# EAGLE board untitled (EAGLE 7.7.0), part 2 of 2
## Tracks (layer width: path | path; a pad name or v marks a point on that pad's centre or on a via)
+5V  (2 unrouted)
  Top 0.406: 32.8,2.1 33.2,2.1 33.2,2.2 | T1.E 32.8,2.12 32.8,2.1 | 32.8,2.1 31.5,2.1 31.5,1.2 28.6,1.2 28.6,4.5 25.2,4.5 24,5.7 19.4,5.7 18.6,6.5 18.6,7.8 17.1,9.3
  Top 0.813: R11.2 16.69,10.01 14.6,12.1 13.52,12.1 D1.C
  Top 1.27: C8.1 8.42,19.82 8,19.4 8,18.2 8.8,17.4 10.52,17.4 D1.C
+5V1  (2 unrouted)
  Top 0.406: 32.8,35.4 33.2,35.4 33.2,35.5 | T2.E 32.8,35.42 32.8,35.4 | 32.8,35.4 31.5,35.4 31.5,34.5 28.6,34.5 28.6,37.8 25.2,37.8 24,39 19.4,39 18.6,39.8 18.6,41.1 17.1,42.6
  Top 0.813: R25.2 16.69,43.31 14.6,45.4 13.52,45.4 D3.C
  Top 1.27: C13.1 8.42,53.12 8,52.7 8,51.5 8.8,50.7 10.52,50.7 D3.C
+5V2  (2 unrouted)
  Top 0.406: 32.8,68.7 33.2,68.7 33.2,68.8 | T3.E 32.8,68.72 32.8,68.7 | 32.8,68.7 31.5,68.7 31.5,67.8 28.6,67.8 28.6,71.1 25.2,71.1 24,72.3 19.4,72.3 18.6,73.1 18.6,74.4 17.1,75.9
  Top 0.813: R39.2 16.69,76.61 14.6,78.7 13.52,78.7 D5.C
  Top 1.27: C20.1 8.42,86.42 8,86 8,84.8 8.8,84 10.52,84 D5.C
N$1  (via drill 0.5)  (12 unrouted)
  Top 0.406: 80,13.29 80,13 | Q1.E 22,1.74 22,1.9 | Q1.E 23.34,0.5 40,0.5 40.6,1.1 40.6,2.2 42.1,0.7 75.7,0.7 75.7,1.5 C6.2 | 14.2,16.7 14.4,16.7 14.4,16.3 | Q1.E 21.8,1.4 20.8,0.5 13.1,0.5 11.4,1.9 11.4,7.2 11.2,7.4 4.89,7.4 X1.2
  Top 1.27: 25.4,17.3 25.4,17.5 21.7,17.5 21.7,17.4 21.6,17.4 21.6,17.5 20.8,17.5 20.8,16.2 21.7,16.2 | R5.2 89.2,13.16 89.2,10.6 70.1,10.6 70.1,13.2 69.8,13.2 69.8,10.6 | 69.8,10.5 69.8,10.6 | 69.8,10.6 70.8,10.6 70.8,11.2 71.1,11.2 71.1,12.2 88.6,12.2 88.6,12.1 87.9,12.1 87.9,11.4 71.9,11.4 71.9,11.2 | D1.A 14.16,17.16 C8.2 14.4,19.82 14.4,16.7 | 14.4,16.3 15.2,16.3 v15.8,18.2 | C2.2 21.7,14.63 21.7,16.1 | 21.7,16.2 v21.7,16.7 v23,16.7 U$1.1 | 15.78,16.7 15.78,17.71 | 21.7,16.2 21.7,16.1 | 21.7,16.1 21.4,16.1 21.4,16.9
  Top 3.81: C5.- 68.9,23.37 68.9,24.4
  Bottom 1.27: 39.5,2 19.4,2 19.4,5.4 36.7,5.4 37.8,4.3 37.8,3 37.5,2.7 20.6,2.7 20.2,3.1 20.2,4 20.4,4.2 36.5,4.2 37.2,3.5 21.3,3.5 21.2,3.4 37.1,3.4 39,1.5 20.1,1.5 | 20.1,1.5 19.4,1.5 | 19.4,1.5 19.4,4.8 18.7,5.5 18.7,16.7 | 18.7,16.7 18.7,20.9 17.6,22 12.9,22 10.2,24.7 10.7,24.7 10.7,27.8 10.5,28 10.5,25.8 10.3,25.6 10.3,25.3 13,22.6 16.4,22.6 | 16.4,22.6 18.5,22.6 18.6,22.5 18.6,21.5 18.4,21.3 | 18.4,21.3 18.7,21.3 | 18.4,21.3 12.6,21.3 10.3,23.6 10.3,21.6 10.8,21.6 12,20.4 15,20.4 15.2,20.6 v15.8,18.2 | v15.8,18.2 15.2,1.5 15.3,1.4 20,1.4 20.1,1.5 | 19.4,1.5 18.8,1.5 18.5,1.8 18.5,4.7 18.6,4.8 | v15.8,18.2 15.7,20.1 15.7,18.1 | v21.7,16.7 v20.5,16.7 | v20.5,16.7 18.7,16.7 | C1.- 16.4,28.3 16.4,22.6 | v20.5,16.7 23.6,16.7 23.6,17.9 19.4,17.9
  Bottom 2.54: 85.2,10.7 86.9,10.7 86.9,9.9 89.6,9.9 89.6,24.1 68.3,24.1 68.3,24.7 68.5,24.7 68.5,22 69.6,22 69.6,20.3 69.5,20.3 69.5,14 42.6,14 42.6,14.3 | 42.4,14.3 42.4,11.2 87.9,11.2 87.9,22.7 71.39,22.7 | 69.3,22.7 71.39,22.7 | 71.39,22.7 R5.2 42.8,13.16 42.8,12.8 43.6,12.8 43.6,5.2 71.8,5.2 | 71.8,5.2 71.8,4.9 | 71.8,5.2 71.8,9.3 45.3,9.3 45.3,10.6 45.8,10.6 45.8,6.6 70.7,6.6 70.7,7.3 47,7.3 47,7.8 72.4,7.8 v72.4,11.1 72.4,21.9 85.6,21.9 85.6,20.7 86.5,20.7 86.5,13.7 74.4,13.7 | 74.4,13.7 74.4,12.89 | 74.4,13.7 74.4,20.7 84.9,20.7 84.9,19.1 85.4,19.1 85.4,14.7 75.6,14.7 75.6,14.5 76.1,14.5 76.1,18.6 83.3,18.6 83.3,18.2 83.5,18.2 83.5,16.4 77.9,16.4 77.9,16.2 83.4,16.2 83.4,4.5 80.4,4.5 | 80.4,4.5 80.4,4.3 | 80.4,4.5 80.4,9.3 81.9,9.3 | 82.5,9.3 81.9,9.3 | 81.9,9.3 81.9,4.9 | 84.7,2.6 85.6,2.6 85.6,1.5 78.3,1.5 78.3,2 78.4,2 78.4,3.1 82.5,3.1 82.5,2.6 78.1,2.6 78.1,3.7 39.5,3.7 39.5,2 73.2,2 73.2,2.4 73,2.4 73,2.6 | X1.2 4.46,7.9 7.9,7.9 8.7,8.7 8.7,32 7.2,32 7.7,31.5 7.7,1.2 8.7,1.2 8.8,1.3 8.8,8.1 8.01,8.89 C4.-
  Bottom 3.81: 84.7,2.6 84.7,2.8 85.2,2.8 85.2,10.7
N$2  (3 unrouted)
  Top 1.27: U$1.3 30.4,13.3 30.4,13.6 30.3,13.6 30.2,18.2 30.2,19.7 | DPAK1.1 31.17,27.4 30.4,27.4 30.4,22.6 30.2,22.6 30.2,20.4 30.2,19.7 | PAD4.1 47,18.2 47,19.7 30.2,19.7
N$3  (3 unrouted)
  Top 1.27: R9.2 2.78,27.11 C4.+ 2.93,28.3 2.9,28.3 2.9,32.4 17.8,32.4 17.8,23.12 | U$1.4 21.74,11.6 | 21.74,11.6 C2.1 | 21.74,11.6 17.8,11.6 17.8,23.12 | R14.2 17.8,23.12
  Bottom 1.016: X1.3 3,2.78 3,4.2 5.2,4.2 5.2,0.6 1.6,0.6 | 1.6,0.6 1.6,0.5 | 1.6,0.6 1.6,1.2 4.5,1.2
  Bottom 1.27: L1.1 64.2,18.2 64.2,17.9 64.3,17.9 64.3,31.8 17.8,31.8 17.8,32.1
  Bottom 2.54: X1.3 1.3,2.78 1.3,32.1 3.5,32.1 3.5,16.8
N$4  (4 unrouted)
  Top 0.406: 71.72,15.63 72,15.63 72,16.2 | X2.2 95.9,24.88 95.9,25.1
  Top 1.27: R6.2 71.72,15.63 R5.1
  Top 2.54: X2.2 98.7,24.88 98.7,23.5 98.6,23.5 98.6,16 71.1,16 71.1,16.5 72,16.5 72,16.2
N$5
  Top 0.406: R7.2 R8.1 44.63,5 46.3,5 48.5,2.8 73.1,2.8 75.65,5.35 C6.1
N$6  (2 unrouted)
  Top 0.406: R7.1 44.3,10.74 44.3,10.9 | 45.35,10.85 46.7,9.5 46.7,7.9 50.1,4.5 69.7,4.5 74.3,8 77.1,8 80.05,5.95 80.05,3.75 80.4,3.4 88.8,3.4 | 45.35,10.85 45.3,10.9 | R6.1 92.38,4.48 91.4,3.5 88.9,3.5 | 45.35,10.85 44.51,10.85 R7.1 | U$1.5 25.6,9.9 25.6,5.3 42.9,5.3 42.9,10.3 44.2,10.3 | D2.A 44.51,13.1 R7.1
N$7  (3 unrouted)
  Top 0.406: 79.5,29.96 79.5,30.79 | D2.C 44.6,15.1 57.1,15.1 57.1,32.4
  Top 1.27: DPAK1.4 40,25.3 40,32.4 57.1,32.4 65.4,32.4 65.4,32.5
  Top 3.81: 78.22,31.02 77.6,30.4 77.6,28.79 C5.+
N$8  (1 unrouted)
  Top 0.406: R11.1 16.69,5.5 17.8,5.5 17.8,4.8 23.6,4.8 23.6,3.1 | Q1.C R12.2
N$9
  Top 0.406: T1.B 32.7,4.02 32.7,3.8 29.96,3.8 R12.1
N$10
  Bottom 1.27: 3.9,6.3 7.8,6.3
N$11  (via drill 0.5)
  other vias: 20.5,17.9
N$12  (via drill 0.5)
  other vias: 21.7,17.9
N$13
  Top 0.406: 35.3,2.9 35.3,3.07 T1.C 35.14,2.8 38.2,2.8 | 38.2,2.8 38.2,2.69 R13.2 38.3,2.69 38.3,4.5 42.2,4.5 42.7,4 42.7,2.5 44.33,2.5 R8.2 | 38.2,2.9 38.2,2.8
N$14
  Top 0.406: R10.2 19.3,2.31 19.3,3.8 21.8,3.8 Q1.B
N$15  (1 unrouted)
  Top 0.406: 15.9,2.7 16,2.8 16,3 15.9,3.1 15.9,4.1 15,5 15,8 14.6,8.4 9.4,12.8 9.4,12.84 X1.1
N$16  (3 unrouted)
  Top 1.27: R23.2 2.78,60.41 C10.+ 2.93,61.6 2.9,61.6 2.9,65.7 17.8,65.7 17.8,56.42 | U$2.4 21.74,44.9 | 21.74,44.9 C7.1 | 21.74,44.9 17.8,44.9 17.8,56.42 | R28.2 17.8,56.42
  Bottom 1.016: X3.3 3,36.08 3,37.5 5.2,37.5 5.2,33.9 1.6,33.9 | 1.6,33.9 1.6,33.8 | 1.6,33.9 1.6,34.5 4.5,34.5
  Bottom 1.27: L2.1 64.2,51.5 64.2,51.2 64.3,51.2 64.3,65.1 17.8,65.1 17.8,65.4
  Bottom 2.54: X3.3 1.3,36.08 1.3,65.4 3.5,65.4 3.5,50.1
N$17  (4 unrouted)
  Top 0.406: 71.72,48.93 72,48.93 72,49.5 | X4.2 95.9,58.18 95.9,58.4
  Top 1.27: R20.2 71.72,48.93 R19.1
  Top 2.54: X4.2 98.7,58.18 98.7,56.8 98.6,56.8 98.6,49.3 71.1,49.3 71.1,49.8 72,49.8 72,49.5
N$18  (via drill 0.5)
  other vias: 23,17.9
N$19
  Top 0.406: R21.2 R22.1 44.63,38.3 46.3,38.3 48.5,36.1 73.1,36.1 75.65,38.65 C12.1
N$20  (1 unrouted)
  Top 0.406: R25.1 16.69,38.8 17.8,38.8 17.8,38.1 23.6,38.1 23.6,36.4 | Q2.C R26.2
N$21
  Top 0.406: 35.3,36.2 35.3,36.37 T2.C 35.14,36.1 38.2,36.1 | 38.2,36.1 38.2,35.99 R27.2 38.3,35.99 38.3,37.8 42.2,37.8 42.7,37.3 42.7,35.8 44.33,35.8 R22.2 | 38.2,36.2 38.2,36.1
N$22  (1 unrouted)
  Top 0.406: 15.9,36 16,36.1 16,36.3 15.9,36.4 15.9,37.4 15,38.3 15,41.3 14.6,41.7 9.4,46.1 9.4,46.14 X3.1
N$23
  Top 0.406: R24.2 19.3,35.61 19.3,37.1 21.8,37.1 Q2.B
N$24
  Top 0.406: T2.B 32.7,37.32 32.7,37.1 29.96,37.1 R26.1
N$25
  Top 1.27: 20.4,16.1 20.3,16.1 20.3,17.9 23.1,17.9 | 23.5,17.9 23.1,17.9 | 23.1,17.9 23.1,16 20.4,16
N$26  (via drill 0.5)
  Top 1.27: 18.6,12.2 18.7,12.2 18.7,32.5 2.2,32.5 2.2,32.4 0.7,32.4 0.7,32.2 0.6,32.2 v0.7,31.4 0.6,26.1 4.1,26.1 4.1,26.3 4.2,26.3 4.2,32.6 v3.1,32.6 v1.9,32.6 v0.7,32.6 0.6,32.6 0.6,32.5 1.8,32.5 v1.9,31.4 1.8,26.9
N$27  (via drill 0.5)
  Top 1.27: 4.7,31.4 v15.6,31.4 v16.8,31.4 17.9,31.4 17.9,31.3 17.6,31.3 17.6,30.2 v16.8,30.2 v15.6,30.2 4,30.2 4,30.5
  Bottom 1.27: 63.1,32.4 63.1,32.6 22.2,32.6 | 22.2,32.4 22.2,32.6 | 22.2,32.6 v18,32.6 v16.8,32.6 15.8,32.6 15.8,31.7 15.9,31.7 | 17.5,31.7 15.9,31.7 | 15.9,31.7 15.9,31 63.2,31 | 64.3,17.2 65.3,17.2 65.3,32.6 63.2,32.6 63.2,31 | 63.2,30.8 63.2,17 | 63.2,31 63.2,30.8 | 63.2,30.8 62.7,30.8 62.7,30.1 15.6,30.1 v15.6,30.2 v15.6,31.4 v15.6,32.6
N$28  (via drill 0.5)
  Top 1.27: 63.4,31.1 40.6,31.1 | 40.6,31.1 40.6,31.6 | 40.6,31.1 40.6,29.8 40.7,29.8 | 64.2,29.8 40.7,29.8 | 40.7,29.8 40.7,27.8 39.1,27.8 39.1,27.9 39.2,27.9 39.2,32.4 38.2,32.4 38.2,32.1 38.1,32.1 38.1,27.9 v35,28 33.8,27.9 33.8,32.6 73.7,32.6 73.7,32.5 35,32.5 35,28.8 37.1,28.8 37.1,31.3 36.1,31.3 | 36.1,31.3 36.1,31.4 | 36.1,31.3 36.1,29.6
N$29
  Top 1.27: 33.8,27.6 33.6,27.6 33.6,22.7 | 33.6,22.7 33.6,22.6 | 33.6,22.6 41.8,22.6 41.8,30.2 43,30.2 43,22.4 44.1,22.4 44.1,30.2 45.2,30.2 45.2,22.4 | 45.2,22.4 33.6,22.4 33.6,22.6 | 33.6,22.7 34.6,22.7 34.6,27.1 35.8,27.1 35.8,23.6 36.8,23.6 36.8,27.1 37,27.1 37,25.9 | 45.2,22.4 65.8,22.4 65.8,28.9 69.7,28.9 69.7,28.8 46.2,28.8 46.2,23.4 64.7,23.4 64.7,27.9 47.1,27.9 47.1,28 47.2,28 47.2,24.5 63.7,24.5 | 63.7,24.5 63.7,24.4 | 63.7,24.5 63.7,26.9 48.1,26.9 48.1,25.5 63,25.5 63,26.2 49,26.2 49,26.1
N$30
  Top 1.27: 45.5,30.5 62.8,30.5
N$31
  Top 1.27: 40.9,31.9 63.2,31.9 63.2,32
N$32
  Top 1.27: 31.6,27.3 31.7,27.3 31.7,23.7 31.4,23.7 31.4,18.9 32,18.9 32,27.4 30.9,27.4 30.9,24.6 29.4,24.6 29.4,27.7 29.3,27.7 29.3,18.6 29,18.6 29,27.8 32,27.8 32,27.7
N$33
  Top 1.27: 32.5,20.3 50.5,20.3 | 50.5,20.3 50.5,20.2 | 50.5,20.2 50.5,19.8 47.7,19.8 47.7,19.6 50.6,19.6 50.6,17 50.7,17 50.7,16.7 46.8,16.7 46.8,16.9 46.6,16.9 46.6,18.6 32.9,18.6 32.9,19.6 32.7,19.6 32.7,20.7 50.5,20.7 50.5,20.3 | 50.5,20.2 39.6,20.2 39.6,16.1 39.4,16.1 39.4,8.2 38.9,8.2 38.9,17.8 28.6,17.8 28.6,6.6 41.7,6.6 41.7,18 40.6,18 40.6,7.4 29.5,7.4 29.5,7.5
N$34
  Top 1.27: 19.3,12.2 23.1,12.2 23.1,10.9 18.2,10.9 18.2,11 17.7,11 17.7,11.2 17.6,11.2 17.6,15.2 17.5,15.2 17.5,29.4
N$35
  Top 1.27: 16.6,29.8 16.6,22.1 16.9,22.1 16.9,22.2
N$36
  Top 1.27: 18.6,32.4 18.8,32.4 18.8,32.5
N$37  (via drill 0.5)
  Top 1.27: 32,27.9 32,32.6 25.7,32.6 25.7,27.5 25.8,27.5 25.8,21.7 v27.1,21.7 28.4,21.7 28.4,21.6 26.7,21.6 26.7,31.6 31.1,31.6 31.1,28.9 27.8,28.9 27.8,22.6 28.4,22.6 v28.4,23 v28.4,24.3 v28.4,25.6 v28.4,26.9 v28.4,28.2 28.4,30.7 27.6,30.7 27.6,29.6 30.2,29.6 30.2,29.7 29.2,29.7 29.2,30.7 30.3,30.7 30.3,30.5
N$38  (via drill 0.5)
  other vias: 3.2,31.4
N$39  (via drill 0.5)
  other vias: 0.7,30.2
N$40  (via drill 0.5)
  other vias: 1.9,30.2
N$41  (via drill 0.5)
  other vias: 3.2,30.2
N$42  (via drill 0.5)
  other vias: 33.5,7.1
N$43  (via drill 0.5)
  other vias: 34.7,7.1
N$44  (via drill 0.5)
  other vias: 18,31.4
N$45  (via drill 0.5)
  other vias: 18.1,30.2
N$46  (via drill 0.5)
  other vias: 28.7,7.1
N$47  (via drill 0.5)
  other vias: 29.9,7.1
N$48  (via drill 0.5)
  other vias: 31.1,7.1
N$49  (via drill 0.5)
  other vias: 32.3,7.1
N$50  (via drill 0.5)
  other vias: 35.9,7.1
N$51  (via drill 0.5)
  other vias: 37.1,7.1
N$52  (via drill 0.5)
  other vias: 38.3,7.1
N$53  (via drill 0.5)
  other vias: 39.5,7.1
N$54  (via drill 0.5)
  other vias: 40.7,7.1
N$55  (via drill 0.5)
  other vias: 39.9,8.4
N$56  (via drill 0.5)
  other vias: 41.2,8.4
N$57  (via drill 0.5)
  other vias: 36.2,22.9
N$58  (via drill 0.5)
  other vias: 40.2,11
N$59  (via drill 0.5)
  other vias: 40.2,12.2
N$60  (via drill 0.5)
  other vias: 40.2,13.5
N$61  (via drill 0.5)
  other vias: 40.2,14.8
N$62  (via drill 0.5)
  other vias: 40.2,16.1
N$63  (via drill 0.5)
  other vias: 40.2,17.4
N$64  (via drill 0.5)
  other vias: 29.2,19.3
N$65  (via drill 0.5)
  other vias: 30.4,19.3
N$66  (via drill 0.5)
  other vias: 31.6,19.3
N$67  (via drill 0.5)
  other vias: 32.8,19.3
N$68  (via drill 0.5)
  other vias: 34,19.3
N$69  (via drill 0.5)
  other vias: 35.2,19.3
N$70  (via drill 0.5)
  other vias: 36.4,19.3
N$71  (via drill 0.5)
  other vias: 37.6,19.3
N$72  (via drill 0.5)
  other vias: 38.8,19.3
N$73  (via drill 0.5)
  other vias: 40,19.3
N$74  (via drill 0.5)
  other vias: 29.2,20.5
N$75  (via drill 0.5)
  other vias: 30.4,20.5
N$76  (via drill 0.5)
  other vias: 31.6,20.5
N$77  (via drill 0.5)
  other vias: 32.8,20.5
N$78  (via drill 0.5)
  other vias: 34,20.5
N$79  (via drill 0.5)
  other vias: 35.2,20.5
N$80  (via drill 0.5)
  other vias: 36.4,20.5
N$81  (via drill 0.5)
  other vias: 37.6,20.5
N$82  (via drill 0.5)
  other vias: 38.8,20.5
N$83
  Top 2.54: 71.4,16.8 96.2,16.8 96.2,25.1 87.3,25.1 87.3,24.9 87.5,24.9 87.5,18.7 94.3,18.7 | 94.5,18.7 94.3,18.7 | 94.3,18.7 94.3,23.3 89.7,23.3 89.7,20.1 93.1,20.1 93.1,20.3 91.9,20.3 91.9,21.7
N$84
  Top 3.81: 88.3,30.7 97.9,30.7 97.9,31 88.4,31 88.4,31.1 64.7,31.1 64.7,31.2
N$85
  Top 2.54: 71.4,50.1 96.2,50.1 96.2,58.4 87.3,58.4 87.3,58.2 87.5,58.2 87.5,52 94.3,52 | 94.5,52 94.3,52 | 94.3,52 94.3,56.6 89.7,56.6 89.7,53.4 93.1,53.4 93.1,53.6 91.9,53.6 91.9,55
N$86
  Top 3.81: 88.3,64 97.9,64 97.9,64.3 88.4,64.3 88.4,64.4 64.7,64.4 64.7,64.5
N$87
  Bottom 2.54: 72.9,41.2 72.9,38.8 72.8,38.8 72.8,43.1 78.4,43.1 78.4,38.6
N$88  (via drill 0.5)
  other vias: 88.1,44.4
N$89  (via drill 0.5)
  other vias: 86.9,44.4
N$90  (via drill 0.5)
  other vias: 85.7,44.4
N$91  (via drill 0.5)
  other vias: 84.5,44.4
N$92  (via drill 0.5)
  other vias: 83.3,44.4
N$93
  Bottom 2.54: 72.9,7.9 72.9,5.5 72.8,5.5 72.8,9.8 78.4,9.8 78.4,5.3
N$94  (via drill 0.5)
  other vias: 88.1,11.1
N$95  (via drill 0.5)
  other vias: 86.9,11.1
N$96  (via drill 0.5)
  other vias: 85.7,11.1
N$97  (via drill 0.5)
  other vias: 84.5,11.1
N$98  (via drill 0.5)
  other vias: 83.3,11.1
N$99  (via drill 0.5)
  other vias: 82.1,11.1
N$100  (via drill 0.5)
  other vias: 80.9,11.1
N$101  (via drill 0.5)
  other vias: 79.7,11.1
N$102  (via drill 0.5)
  other vias: 78.5,11.1
N$103  (via drill 0.5)
  other vias: 77.3,11.1
N$104  (via drill 0.5)
  other vias: 76,11.1
N$105  (via drill 0.5)
  other vias: 74.8,11.1
N$106  (via drill 0.5)
  other vias: 73.6,11.1
N$107  (via drill 0.5)
  other vias: 71.2,11.1
N$108  (via drill 0.5)
  other vias: 69.9,11.1
N$109  (via drill 0.5)
  other vias: 67.9,23.6
N$110  (via drill 0.5)
  other vias: 69.2,23.6
N$111  (via drill 0.5)
  other vias: 70.5,23.6
N$112  (via drill 0.5)
  other vias: 71.8,23.6
N$113  (via drill 0.5)
  other vias: 73.1,23.6
N$114  (via drill 0.5)
  other vias: 74.4,23.6
N$115  (via drill 0.5)
  other vias: 74.4,22.3
N$116  (via drill 0.5)
  other vias: 73.1,22.3
N$117  (via drill 0.5)
  other vias: 71.7,22.3
N$118  (via drill 0.5)
  other vias: 70.4,22.3
N$119  (via drill 0.5)
  other vias: 69.1,22.3
N$120  (via drill 0.5)
  other vias: 67.9,22.4
N$121  (via drill 0.5)
  other vias: 82.1,44.4
N$122  (via drill 0.5)
  other vias: 80.9,44.4
N$123  (via drill 0.5)
  other vias: 79.7,44.4
N$124  (via drill 0.5)
  other vias: 78.5,44.4
N$125  (via drill 0.5)
  other vias: 77.3,44.4
N$126  (via drill 0.5)
  other vias: 76,44.4
N$127  (via drill 0.5)
  other vias: 74.8,44.4
N$128  (via drill 0.5)
  other vias: 73.6,44.4
N$129  (via drill 0.5)
  other vias: 40,20.6
N$130
  Bottom 1.27: 18.1,2.2 16,2.2 16,20.7 | 16,20.7 16.7,20.7 | 16.7,20.7 17.8,20.7 17.8,2.9 17,2.9 17,3.1 16.8,3.1 16.8,20.4 16.7,20.4 16.7,20.7 | 16,20.7 10.3,20.7 10.3,25.1 10.2,25.1 10.2,28 9.8,28 9.8,25.6
N$131
  Top 1.27: 14.6,16 15.8,16 15.8,20.1 15.1,20.1 | 15,20.1 15.1,20.1 | 15.1,20.1 15.1,17.6 14.2,17.6 14.2,16
N$132  (via drill 0.5)
  other vias: 71.2,44.4
N$133  (via drill 0.5)
  other vias: 41.2,20.5
N$134  (4 unrouted)
  Top 0.406: 25.9,14.9 25.9,15 27.1,15 27.1,20.28 R14.1 24,20.28 24,28.2
  Top 1.27: U$1.2 25.1,15
N$135  (via drill 0.5)
  other vias: 41.2,19.3
N$136  (via drill 0.5)
  other vias: 41.4,17.8
N$137  (via drill 0.5)
  other vias: 41.5,16.5
N$138  (via drill 0.5)
  other vias: 28.4,21.8
N$139  (via drill 0.5)
  other vias: 27.1,28.2
N$140  (via drill 0.5)
  other vias: 27.1,27
N$141  (via drill 0.5)
  other vias: 27.1,25.6
N$142  (via drill 0.5)
  other vias: 27.1,24.3
N$143  (via drill 0.5)
  other vias: 27.1,22.9
N$144  (via drill 0.5)
  other vias: 42.5,22.7
N$145  (via drill 0.5)
  other vias: 42.5,24
N$146  (via drill 0.5)
  other vias: 42.5,25.3
N$147  (via drill 0.5)
  other vias: 42.5,26.6
N$148  (via drill 0.5)
  other vias: 42.5,27.9
N$149  (via drill 0.5)
  other vias: 43.8,27.9
N$150  (via drill 0.5)
  other vias: 69.9,44.4
N$151  (via drill 0.5)
  other vias: 43.8,26.6
N$152  (via drill 0.5)
  other vias: 43.7,25.3
N$153  (via drill 0.5)
  other vias: 43.7,24
N$154  (via drill 0.5)
  other vias: 43.7,22.7
N$155  (via drill 0.5)
  Bottom 1.27: 34,28.4 v37.5,28.4 v38.7,28.4 v40.1,28.4 v41.3,28.4 61.4,28.4 61.4,22.4 33.9,22.4 33.9,28.4 34.7,28.4 34.7,23
N$156
  Bottom 1.27: 35.3,23.2 60.6,23.2 60.6,27.4 35.6,27.4 35.6,24.3 59.7,24.3 59.7,26.5 36.6,26.5 36.6,25.3
N$157
  Bottom 1.27: 37.3,25.2 59.2,25.2 59.2,25.5 37.6,25.5 37.6,26.2
N$158  (via drill 0.5)
  Bottom 1.27: 25.8,28.2 25.7,28.2 | 25.7,28.2 25.7,28.3 | 25.7,28.3 25.7,28.5 32,28.5 32,20.2 32.8,20.2 32.8,20.7 50.5,20.7 50.5,20.4 50.6,20.4 50.6,16.7 41.7,16.7 41.7,17.5 41.4,17.5 41.4,19.9 49.7,19.9 49.7,19.4 42.7,19.4 42.7,17.5 49.6,17.5 49.6,18.6 43.7,18.6 43.7,18.5 40.5,18.5 40.5,15.8 40.3,15.8 40.3,15.1 40.1,15.1 v40.1,9.7 40.1,8.9 41.3,8.9 41.3,7.1 25.7,7.1 25.7,28.2 | 25.7,28.3 31,28.3 31,20.1 26.3,20.1 26.3,20.8 26.5,20.8 26.5,27.7 30.1,27.7 30.1,21.1 27.4,21.1 27.4,27.2 29,27.2 29,21.6 28.1,21.6 28.1,26.5
N$159
  Bottom 1.27: 26.4,19.1 40.8,19.1 40.8,19.9 34,19.9 34,19.8 39.3,19.8 39.3,7.3 40.3,7.3 40.3,7.9 26.8,7.9 26.8,18.2 39,18.2 39,8.4 27.5,8.4 27.5,17.3 37.9,17.3 37.9,9.1 28.5,9.1 28.5,16.3 36.8,16.3 36.8,10 29.4,10 29.4,15.4 35.6,15.4 35.6,10.8 30.3,10.8 30.3,14.7 34.5,14.7 34.5,11.8 31.3,11.8 31.3,13.7 33.5,13.7 33.5,12.6 32.2,12.6 32.2,12.8
N$160
  Bottom 1.27: 37.5,5 43,5 43,5.1 42.5,5.1 | 42.5,5.1 37,5.1 | 37,5.1 37,5.3 42.5,5.3 42.5,5.1 | 37,5.1 19.3,5.1 19.3,23 12.1,23 12.1,22.9
N$161
  Top 0.406: 23.6,28.3 23.7,28.3 23.7,20.6 22.8,20.6
N$162
  Bottom 0.406: 25.6,6.7 20.5,6.7 20.5,15.3 25.1,15.3 25.1,7 20.8,7 20.8,15.1 24.8,15.1 24.8,14.8 24.7,14.8 24.7,7.3 21.2,7.3 21.2,7.4 21,7.4 21,14.9 24.4,14.9 24.4,7.7 21.3,7.7 21.3,14.7 24,14.7 24,8 21.6,8 21.6,14.5 23.7,14.5 23.7,8.3 21.9,8.3 21.9,14.3 23.4,14.3 23.4,8.4 22.3,8.4 22.3,14 23.1,14 23.1,8.7 22.7,8.7 22.7,13.8 22.4,13.8 22.4,13.1
N$163
  Bottom 0.406: 25.3,19.3 25,19.3 25,15.6 24.9,15.6 24.9,19.2 20.6,19.2 20.6,20 20.7,20 20.7,26.6 25.1,26.6 25.1,26.1 24.9,26.1 24.9,26.4 25,26.4 25,19.5 20.9,19.5 20.9,19.8 21,19.8 21,26.2 24.7,26.2 24.7,19.8 21.3,19.8 21.3,25.8 24.4,25.8 24.4,20.1 21.7,20.1 21.7,25.5 24,25.5 24,20.3 22.1,20.3 22.1,25.2 23.7,25.2 23.7,20.6 22.5,20.6 22.5,24.9 23.4,24.9 23.4,20.8 22.9,20.8 22.9,24.6
N$164  (via drill 0.5)
  other vias: 36.2,24.2
N$165  (via drill 0.5)
  other vias: 36.2,25.5
N$166  (via drill 0.5)
  other vias: 36.3,26.7
N$167  (via drill 0.5)
  other vias: 36.3,28
N$168  (via drill 0.5)
  other vias: 34.8,22.9
N$169  (via drill 0.5)
  other vias: 34.8,24.2
N$170  (via drill 0.5)
  other vias: 34.9,25.5
N$171  (via drill 0.5)
  other vias: 35,26.7
N$172  (via drill 0.5)
  other vias: 67.9,56.9
N$173  (via drill 0.5)
  other vias: 69.2,56.9
N$174  (via drill 0.5)
  other vias: 70.5,56.9
N$175  (via drill 0.5)
  other vias: 71.8,56.9
N$176  (via drill 0.5)
  other vias: 73.1,56.9
N$177  (via drill 0.5)
  other vias: 74.4,56.9
N$178  (via drill 0.5)
  other vias: 74.4,55.6
N$179  (via drill 0.5)
  other vias: 73.1,55.6
N$180  (via drill 0.5)
  other vias: 71.7,55.6
N$181  (via drill 0.5)
  other vias: 70.4,55.6
N$182  (via drill 0.5)
  other vias: 69.1,55.6
N$183  (via drill 0.5)
  other vias: 67.9,55.7
N$184
  Bottom 1.27: 3.9,39.6 7.8,39.6
N$185
  Bottom 1.27: 18.1,35.5 16,35.5 16,54 | 16,54 16.7,54 | 16.7,54 17.8,54 17.8,36.2 17,36.2 17,36.4 16.8,36.4 16.8,53.7 16.7,53.7 16.7,54 | 16,54 10.3,54 10.3,58.4 10.2,58.4 10.2,61.3 9.8,61.3 9.8,58.9
N$186
  Top 1.27: 14.6,49.3 15.8,49.3 15.8,53.4 15.1,53.4 | 15,53.4 15.1,53.4 | 15.1,53.4 15.1,50.9 14.2,50.9 14.2,49.3
N$187  (3 unrouted)
  Top 1.27: U$2.3 30.4,46.6 30.4,46.9 30.3,46.9 30.2,51.5 30.2,53 | DPAK2.1 31.17,60.7 30.4,60.7 30.4,55.9 30.2,55.9 30.2,53.7 30.2,53 | PAD2.1 47,51.5 47,53 30.2,53
N$188  (4 unrouted)
  Top 0.406: 25.9,48.2 25.9,48.3 27.1,48.3 27.1,53.58 R28.1 24,53.58 24,61.5
  Top 1.27: U$2.2 25.1,48.3
N$189  (3 unrouted)
  Top 0.406: X4.1 79.5,63.26 79.5,64.09 | D4.C 44.6,48.4 57.1,48.4 57.1,65.7
  Top 1.27: DPAK2.4 40,58.6 40,65.7 57.1,65.7 65.4,65.7 65.4,65.8
  Top 3.81: 78.22,64.32 77.6,63.7 77.6,62.09 C11.+
N$190  (2 unrouted)
  Top 0.406: R21.1 44.3,44.04 44.3,44.2 | 45.35,44.15 46.7,42.8 46.7,41.2 50.1,37.8 69.7,37.8 74.3,41.3 77.1,41.3 80.05,39.25 80.05,37.05 80.4,36.7 88.8,36.7 | 45.35,44.15 45.3,44.2 | R20.1 92.38,37.78 91.4,36.8 88.9,36.8 | 45.35,44.15 44.51,44.15 R21.1 | U$2.5 25.6,43.2 25.6,38.6 42.9,38.6 42.9,43.6 44.2,43.6 | D4.A 44.51,46.4 R21.1
N$191  (via drill 0.5)  (12 unrouted)
  Top 0.406: 80,46.59 80,46.3 | Q2.E 22,35.04 22,35.2 | Q2.E 23.34,33.8 40,33.8 40.6,34.4 40.6,35.5 42.1,34 75.7,34 75.7,34.8 C12.2 | 14.2,50 14.4,50 14.4,49.6 | Q2.E 21.8,34.7 20.8,33.8 13.1,33.8 11.4,35.2 11.4,40.5 11.2,40.7 4.89,40.7 X3.2
  Top 1.27: 25.4,50.6 25.4,50.8 21.7,50.8 21.7,50.7 21.6,50.7 21.6,50.8 20.8,50.8 20.8,49.5 21.7,49.5 | R19.2 89.2,46.46 89.2,43.9 70.1,43.9 70.1,46.5 69.8,46.5 69.8,43.9 | 69.8,43.8 69.8,43.9 | 69.8,43.9 70.8,43.9 70.8,44.5 71.1,44.5 71.1,45.5 88.6,45.5 88.6,45.4 87.9,45.4 87.9,44.7 71.9,44.7 71.9,44.5 | D3.A 14.16,50.46 C13.2 14.4,53.12 14.4,50 | 14.4,49.6 15.2,49.6 v15.8,51.5 | C7.2 21.7,47.93 21.7,49.4 | 21.7,49.5 v21.7,50 v23,50 U$2.1 | 15.78,50 15.78,51.01 | 21.7,49.5 21.7,49.4 | 21.7,49.4 21.4,49.4 21.4,50.2
  Top 3.81: C11.- 68.9,56.67 68.9,57.7
  Bottom 1.27: 39.5,35.3 19.4,35.3 19.4,38.7 36.7,38.7 37.8,37.6 37.8,36.3 37.5,36 20.6,36 20.2,36.4 20.2,37.3 20.4,37.5 36.5,37.5 37.2,36.8 21.3,36.8 21.2,36.7 37.1,36.7 39,34.8 20.1,34.8 | 20.1,34.8 19.4,34.8 | 19.4,34.8 19.4,38.1 18.7,38.8 18.7,50 | 18.7,50 18.7,54.2 17.6,55.3 12.9,55.3 10.2,58 10.7,58 10.7,61.1 10.5,61.3 10.5,59.1 10.3,58.9 10.3,58.6 13,55.9 16.4,55.9 | 16.4,55.9 18.5,55.9 18.6,55.8 18.6,54.8 18.4,54.6 | 18.4,54.6 18.7,54.6 | 18.4,54.6 12.6,54.6 10.3,56.9 10.3,54.9 10.8,54.9 12,53.7 15,53.7 15.2,53.9 v15.8,51.5 | v15.8,51.5 15.2,34.8 15.3,34.7 20,34.7 20.1,34.8 | 19.4,34.8 18.8,34.8 18.5,35.1 18.5,38 18.6,38.1 | v15.8,51.5 15.7,53.4 15.7,51.4 | v21.7,50 v20.5,50 | v20.5,50 18.7,50 | C14.- 16.4,61.6 16.4,55.9 | v20.5,50 23.6,50 23.6,51.2 19.4,51.2
  Bottom 2.54: 85.2,44 86.9,44 86.9,43.2 89.6,43.2 89.6,57.4 68.3,57.4 68.3,58 68.5,58 68.5,55.3 69.6,55.3 69.6,53.6 69.5,53.6 69.5,47.3 42.6,47.3 42.6,47.6 | 42.4,47.6 42.4,44.5 87.9,44.5 87.9,56 71.39,56 | 69.3,56 71.39,56 | 71.39,56 R19.2 42.8,46.46 42.8,46.1 43.6,46.1 43.6,38.5 71.8,38.5 | 71.8,38.5 71.8,38.2 | 71.8,38.5 71.8,42.6 45.3,42.6 45.3,43.9 45.8,43.9 45.8,39.9 70.7,39.9 70.7,40.6 47,40.6 47,41.1 72.4,41.1 v72.4,44.4 72.4,55.2 85.6,55.2 85.6,54 86.5,54 86.5,47 74.4,47 | 74.4,47 74.4,46.19 | 74.4,47 74.4,54 84.9,54 84.9,52.4 85.4,52.4 85.4,48 75.6,48 75.6,47.8 76.1,47.8 76.1,51.9 83.3,51.9 83.3,51.5 83.5,51.5 83.5,49.7 77.9,49.7 77.9,49.5 83.4,49.5 83.4,37.8 80.4,37.8 | 80.4,37.8 80.4,37.6 | 80.4,37.8 80.4,42.6 81.9,42.6 | 82.5,42.6 81.9,42.6 | 81.9,42.6 81.9,38.2 | 84.7,35.9 85.6,35.9 85.6,34.8 78.3,34.8 78.3,35.3 78.4,35.3 78.4,36.4 82.5,36.4 82.5,35.9 78.1,35.9 78.1,37 39.5,37 39.5,35.3 73.2,35.3 73.2,35.7 73,35.7 73,35.9
  Bottom 3.81: 84.7,35.9 84.7,36.1 85.2,36.1 85.2,44
N$192  (via drill 0.5)
  other vias: 20.5,51.2
N$193  (via drill 0.5)
  other vias: 21.7,51.2
N$194  (via drill 0.5)
  other vias: 23,51.2
N$195
  Top 1.27: 20.4,49.4 20.3,49.4 20.3,51.2 23.1,51.2 | 23.5,51.2 23.1,51.2 | 23.1,51.2 23.1,49.3 20.4,49.3
N$196  (via drill 0.5)
  Top 1.27: 18.6,45.5 18.7,45.5 18.7,65.8 2.2,65.8 2.2,65.7 0.7,65.7 0.7,65.5 0.6,65.5 v0.7,64.7 0.6,59.4 4.1,59.4 4.1,59.6 4.2,59.6 4.2,65.9 v3.1,65.9 v1.9,65.9 v0.7,65.9 0.6,65.9 0.6,65.8 1.8,65.8 v1.9,64.7 1.8,60.2
N$197  (via drill 0.5)
  Top 1.27: 4.7,64.7 v15.6,64.7 v16.8,64.7 17.9,64.7 17.9,64.6 17.6,64.6 17.6,63.5 v16.8,63.5 v15.6,63.5 4,63.5 4,63.8
  Bottom 1.27: 63.1,65.7 63.1,65.9 22.2,65.9 | 22.2,65.7 22.2,65.9 | 22.2,65.9 v18,65.9 v16.8,65.9 15.8,65.9 15.8,65 15.9,65 | 17.5,65 15.9,65 | 15.9,65 15.9,64.3 63.2,64.3 | 64.3,50.5 65.3,50.5 65.3,65.9 63.2,65.9 63.2,64.3 | 63.2,64.1 63.2,50.3 | 63.2,64.3 63.2,64.1 | 63.2,64.1 62.7,64.1 62.7,63.4 15.6,63.4 v15.6,63.5 v15.6,64.7 v15.6,65.9
N$198  (via drill 0.5)
  Top 1.27: 63.4,64.4 40.6,64.4 | 40.6,64.4 40.6,64.9 | 40.6,64.4 40.6,63.1 40.7,63.1 | 64.2,63.1 40.7,63.1 | 40.7,63.1 40.7,61.1 39.1,61.1 39.1,61.2 39.2,61.2 39.2,65.7 38.2,65.7 38.2,65.4 38.1,65.4 38.1,61.2 v35,61.3 33.8,61.2 33.8,65.9 73.7,65.9 73.7,65.8 35,65.8 35,62.1 37.1,62.1 37.1,64.6 36.1,64.6 | 36.1,64.6 36.1,64.7 | 36.1,64.6 36.1,62.9
N$199
  Top 1.27: 33.8,60.9 33.6,60.9 33.6,56 | 33.6,56 33.6,55.9 | 33.6,55.9 41.8,55.9 41.8,63.5 43,63.5 43,55.7 44.1,55.7 44.1,63.5 45.2,63.5 45.2,55.7 | 45.2,55.7 33.6,55.7 33.6,55.9 | 33.6,56 34.6,56 34.6,60.4 35.8,60.4 35.8,56.9 36.8,56.9 36.8,60.4 37,60.4 37,59.2 | 45.2,55.7 65.8,55.7 65.8,62.2 69.7,62.2 69.7,62.1 46.2,62.1 46.2,56.7 64.7,56.7 64.7,61.2 47.1,61.2 47.1,61.3 47.2,61.3 47.2,57.8 63.7,57.8 | 63.7,57.8 63.7,57.7 | 63.7,57.8 63.7,60.2 48.1,60.2 48.1,58.8 63,58.8 63,59.5 49,59.5 49,59.4
N$200
  Top 1.27: 45.5,63.8 62.8,63.8
N$201
  Top 1.27: 40.9,65.2 63.2,65.2 63.2,65.3
N$202
  Top 1.27: 31.6,60.6 31.7,60.6 31.7,57 31.4,57 31.4,52.2 32,52.2 32,60.7 30.9,60.7 30.9,57.9 29.4,57.9 29.4,61 29.3,61 29.3,51.9 29,51.9 29,61.1 32,61.1 32,61
N$203
  Top 1.27: 32.5,53.6 50.5,53.6 | 50.5,53.6 50.5,53.5 | 50.5,53.5 50.5,53.1 47.7,53.1 47.7,52.9 50.6,52.9 50.6,50.3 50.7,50.3 50.7,50 46.8,50 46.8,50.2 46.6,50.2 46.6,51.9 32.9,51.9 32.9,52.9 32.7,52.9 32.7,54 50.5,54 50.5,53.6 | 50.5,53.5 39.6,53.5 39.6,49.4 39.4,49.4 39.4,41.5 38.9,41.5 38.9,51.1 28.6,51.1 28.6,39.9 41.7,39.9 41.7,51.3 40.6,51.3 40.6,40.7 29.5,40.7 29.5,40.8
N$204
  Top 1.27: 19.3,45.5 23.1,45.5 23.1,44.2 18.2,44.2 18.2,44.3 17.7,44.3 17.7,44.5 17.6,44.5 17.6,48.5 17.5,48.5 17.5,62.7
N$205
  Top 1.27: 16.6,63.1 16.6,55.4 16.9,55.4 16.9,55.5
N$206
  Top 1.27: 18.6,65.7 18.8,65.7 18.8,65.8
N$207  (via drill 0.5)
  Top 1.27: 32,61.2 32,65.9 25.7,65.9 25.7,60.8 25.8,60.8 25.8,55 v27.1,55 28.4,55 28.4,54.9 26.7,54.9 26.7,64.9 31.1,64.9 31.1,62.2 27.8,62.2 27.8,55.9 28.4,55.9 v28.4,56.3 v28.4,57.6 v28.4,58.9 v28.4,60.2 v28.4,61.5 28.4,64 27.6,64 27.6,62.9 30.2,62.9 30.2,63 29.2,63 29.2,64 30.3,64 30.3,63.8
N$208  (via drill 0.5)
  other vias: 3.2,64.7
N$209  (via drill 0.5)
  other vias: 0.7,63.5
N$210  (via drill 0.5)
  other vias: 1.9,63.5
N$211  (via drill 0.5)
  other vias: 3.2,63.5
N$212  (via drill 0.5)
  other vias: 18,64.7
N$213  (via drill 0.5)
  other vias: 18.1,63.5
N$214  (via drill 0.5)
  other vias: 28.7,40.4
N$215  (via drill 0.5)
  other vias: 29.9,40.4
N$216  (via drill 0.5)
  other vias: 31.1,40.4
N$217  (via drill 0.5)
  other vias: 32.3,40.4
N$218  (via drill 0.5)
  other vias: 33.5,40.4
N$219  (via drill 0.5)
  other vias: 34.7,40.4
N$220  (via drill 0.5)
  other vias: 35.9,40.4
N$221  (via drill 0.5)
  other vias: 37.1,40.4
N$222  (via drill 0.5)
  other vias: 38.3,40.4
N$223  (via drill 0.5)
  other vias: 39.5,40.4
N$224  (via drill 0.5)
  other vias: 40.7,40.4
N$225  (via drill 0.5)
  other vias: 39.9,41.7
N$226  (via drill 0.5)
  other vias: 41.2,41.7
N$227  (via drill 0.5)
  other vias: 40.2,44.3
N$228  (via drill 0.5)
  other vias: 40.2,45.5
N$229  (via drill 0.5)
  other vias: 40.2,46.8
N$230  (via drill 0.5)
  other vias: 40.2,48.1
N$231  (via drill 0.5)
  other vias: 40.2,49.4
N$232  (via drill 0.5)
  other vias: 40.2,50.7
N$233  (via drill 0.5)
  other vias: 29.2,52.6
N$234  (via drill 0.5)
  other vias: 30.4,52.6
N$235  (via drill 0.5)
  other vias: 31.6,52.6
N$236  (via drill 0.5)
  other vias: 32.8,52.6
N$237  (via drill 0.5)
  other vias: 34,52.6
N$238  (via drill 0.5)
  other vias: 35.2,52.6
N$239  (via drill 0.5)
  other vias: 36.4,52.6
N$240  (via drill 0.5)
  other vias: 37.6,52.6
N$241  (via drill 0.5)
  other vias: 38.8,52.6
N$242  (via drill 0.5)
  other vias: 40,52.6
N$243  (via drill 0.5)
  other vias: 29.2,53.8
N$244  (via drill 0.5)
  other vias: 30.4,53.8
N$245  (via drill 0.5)
  other vias: 31.6,53.8
N$246  (via drill 0.5)
  other vias: 32.8,53.8
N$247  (via drill 0.5)
  other vias: 34,53.8
N$248  (via drill 0.5)
  other vias: 35.2,53.8
N$249  (via drill 0.5)
  other vias: 36.4,53.8
N$250  (via drill 0.5)
  other vias: 37.6,53.8
N$251  (via drill 0.5)
  other vias: 38.8,53.8
N$252  (via drill 0.5)
  other vias: 40,53.9
N$253  (via drill 0.5)
  other vias: 41.2,53.8
N$254  (via drill 0.5)
  other vias: 41.2,52.6
N$255  (via drill 0.5)
  other vias: 41.4,51.1
N$256  (via drill 0.5)
  other vias: 41.5,49.8
N$257  (via drill 0.5)
  other vias: 28.4,55.1
N$258  (via drill 0.5)
  other vias: 27.1,61.5
N$259  (via drill 0.5)
  other vias: 27.1,60.3
N$260  (via drill 0.5)
  other vias: 27.1,58.9
N$261  (via drill 0.5)
  other vias: 27.1,57.6
N$262  (via drill 0.5)
  other vias: 27.1,56.2
N$263  (via drill 0.5)
  other vias: 42.5,56
N$264  (via drill 0.5)
  other vias: 42.5,57.3
N$265  (via drill 0.5)
  other vias: 42.5,58.6
N$266  (via drill 0.5)
  other vias: 42.5,59.9
N$267  (via drill 0.5)
  other vias: 42.5,61.2
N$268  (via drill 0.5)
  other vias: 43.8,61.2
N$269  (via drill 0.5)
  other vias: 43.8,59.9
N$270  (via drill 0.5)
  other vias: 43.7,58.6
N$271  (via drill 0.5)
  other vias: 43.7,57.3
N$272  (via drill 0.5)
  other vias: 43.7,56
N$273  (via drill 0.5)
  Bottom 1.27: 34,61.7 v37.5,61.7 v38.7,61.7 v40.1,61.7 v41.3,61.7 61.4,61.7 61.4,55.7 33.9,55.7 33.9,61.7 34.7,61.7 34.7,56.3
N$274
  Bottom 1.27: 35.3,56.5 60.6,56.5 60.6,60.7 35.6,60.7 35.6,57.6 59.7,57.6 59.7,59.8 36.6,59.8 36.6,58.6
N$275
  Bottom 1.27: 37.3,58.5 59.2,58.5 59.2,58.8 37.6,58.8 37.6,59.5
N$276  (via drill 0.5)
  Bottom 1.27: 25.8,61.5 25.7,61.5 | 25.7,61.5 25.7,61.6 | 25.7,61.6 25.7,61.8 32,61.8 32,53.5 32.8,53.5 32.8,54 50.5,54 50.5,53.7 50.6,53.7 50.6,50 41.7,50 41.7,50.8 41.4,50.8 41.4,53.2 49.7,53.2 49.7,52.7 42.7,52.7 42.7,50.8 49.6,50.8 49.6,51.9 43.7,51.9 43.7,51.8 40.5,51.8 40.5,49.1 40.3,49.1 40.3,48.4 40.1,48.4 v40.1,43 40.1,42.2 41.3,42.2 41.3,40.4 25.7,40.4 25.7,61.5 | 25.7,61.6 31,61.6 31,53.4 26.3,53.4 26.3,54.1 26.5,54.1 26.5,61 30.1,61 30.1,54.4 27.4,54.4 27.4,60.5 29,60.5 29,54.9 28.1,54.9 28.1,59.8
N$277
  Bottom 1.27: 26.4,52.4 40.8,52.4 40.8,53.2 34,53.2 34,53.1 39.3,53.1 39.3,40.6 40.3,40.6 40.3,41.2 26.8,41.2 26.8,51.5 39,51.5 39,41.7 27.5,41.7 27.5,50.6 37.9,50.6 37.9,42.4 28.5,42.4 28.5,49.6 36.8,49.6 36.8,43.3 29.4,43.3 29.4,48.7 35.6,48.7 35.6,44.1 30.3,44.1 30.3,48 34.5,48 34.5,45.1 31.3,45.1 31.3,47 33.5,47 33.5,45.9 32.2,45.9 32.2,46.1
N$278
  Bottom 1.27: 37.5,38.3 43,38.3 43,38.4 42.5,38.4 | 42.5,38.4 37,38.4 | 37,38.4 37,38.6 42.5,38.6 42.5,38.4 | 37,38.4 19.3,38.4 19.3,56.3 12.1,56.3 12.1,56.2
N$279
  Top 0.406: 23.6,61.6 23.7,61.6 23.7,53.9 22.8,53.9
N$280
  Bottom 0.406: 25.6,40 20.5,40 20.5,48.6 25.1,48.6 25.1,40.3 20.8,40.3 20.8,48.4 24.8,48.4 24.8,48.1 24.7,48.1 24.7,40.6 21.2,40.6 21.2,40.7 21,40.7 21,48.2 24.4,48.2 24.4,41 21.3,41 21.3,48 24,48 24,41.3 21.6,41.3 21.6,47.8 23.7,47.8 23.7,41.6 21.9,41.6 21.9,47.6 23.4,47.6 23.4,41.7 22.3,41.7 22.3,47.3 23.1,47.3 23.1,42 22.7,42 22.7,47.1 22.4,47.1 22.4,46.4
N$281
  Bottom 0.406: 25.3,52.6 25,52.6 25,48.9 24.9,48.9 24.9,52.5 20.6,52.5 20.6,53.3 20.7,53.3 20.7,59.9 25.1,59.9 25.1,59.4 24.9,59.4 24.9,59.7 25,59.7 25,52.8 20.9,52.8 20.9,53.1 21,53.1 21,59.5 24.7,59.5 24.7,53.1 21.3,53.1 21.3,59.1 24.4,59.1 24.4,53.4 21.7,53.4 21.7,58.8 24,58.8 24,53.6 22.1,53.6 22.1,58.5 23.7,58.5 23.7,53.9 22.5,53.9 22.5,58.2 23.4,58.2 23.4,54.1 22.9,54.1 22.9,57.9
N$282  (via drill 0.5)
  other vias: 36.2,56.2
N$283  (via drill 0.5)
  other vias: 36.2,57.5
N$284  (via drill 0.5)
  other vias: 36.2,58.8
N$285  (via drill 0.5)
  other vias: 36.3,60
N$286  (via drill 0.5)
  other vias: 36.3,61.3
N$287  (via drill 0.5)
  other vias: 34.8,56.2
N$288  (via drill 0.5)
  other vias: 34.8,57.5
N$289  (via drill 0.5)
  other vias: 34.9,58.8
N$290  (via drill 0.5)
  other vias: 35,60
N$291  (3 unrouted)
  Top 1.27: R37.2 2.78,93.71 C17.+ 2.93,94.9 2.9,94.9 2.9,99 17.8,99 17.8,89.72 | U$3.4 21.74,78.2 | 21.74,78.2 C15.1 | 21.74,78.2 17.8,78.2 17.8,89.72 | R42.2 17.8,89.72
  Bottom 1.016: X5.3 3,69.38 3,70.8 5.2,70.8 5.2,67.2 1.6,67.2 | 1.6,67.2 1.6,67.1 | 1.6,67.2 1.6,67.8 4.5,67.8
  Bottom 1.27: L3.1 64.2,84.8 64.2,84.5 64.3,84.5 64.3,98.4 17.8,98.4 17.8,98.7
  Bottom 2.54: X5.3 1.3,69.38 1.3,98.7 3.5,98.7 3.5,83.4
N$292  (4 unrouted)
  Top 0.406: 71.72,82.23 72,82.23 72,82.8 | X6.2 95.9,91.48 95.9,91.7
  Top 1.27: R34.2 71.72,82.23 R33.1
  Top 2.54: X6.2 98.7,91.48 98.7,90.1 98.6,90.1 98.6,82.6 71.1,82.6 71.1,83.1 72,83.1 72,82.8
N$293
  Top 0.406: R35.2 R36.1 44.63,71.6 46.3,71.6 48.5,69.4 73.1,69.4 75.65,71.95 C19.1
N$294  (1 unrouted)
  Top 0.406: R39.1 16.69,72.1 17.8,72.1 17.8,71.4 23.6,71.4 23.6,69.7 | Q3.C R40.2
N$295
  Top 0.406: 35.3,69.5 35.3,69.67 T3.C 35.14,69.4 38.2,69.4 | 38.2,69.4 38.2,69.29 R41.2 38.3,69.29 38.3,71.1 42.2,71.1 42.7,70.6 42.7,69.1 44.33,69.1 R36.2 | 38.2,69.5 38.2,69.4
N$296  (1 unrouted)
  Top 0.406: 15.9,69.3 16,69.4 16,69.6 15.9,69.7 15.9,70.7 15,71.6 15,74.6 14.6,75 9.4,79.4 9.4,79.44 X5.1
N$297
  Top 0.406: R38.2 19.3,68.91 19.3,70.4 21.8,70.4 Q3.B
N$298
  Top 0.406: T3.B 32.7,70.62 32.7,70.4 29.96,70.4 R40.1
N$299
  Top 2.54: 71.4,83.4 96.2,83.4 96.2,91.7 87.3,91.7 87.3,91.5 87.5,91.5 87.5,85.3 94.3,85.3 | 94.5,85.3 94.3,85.3 | 94.3,85.3 94.3,89.9 89.7,89.9 89.7,86.7 93.1,86.7 93.1,86.9 91.9,86.9 91.9,88.3
N$300
  Top 3.81: 88.3,97.3 97.9,97.3 97.9,97.6 88.4,97.6 88.4,97.7 64.7,97.7 64.7,97.8
N$301
  Bottom 2.54: 72.9,74.5 72.9,72.1 72.8,72.1 72.8,76.4 78.4,76.4 78.4,71.9
N$302  (via drill 0.5)
  other vias: 88.1,77.7
N$303  (via drill 0.5)
  other vias: 86.9,77.7
N$304  (via drill 0.5)
  other vias: 85.7,77.7
N$305  (via drill 0.5)
  other vias: 84.5,77.7
N$306  (via drill 0.5)
  other vias: 83.3,77.7
N$307  (via drill 0.5)
  other vias: 82.1,77.7
N$308  (via drill 0.5)
  other vias: 80.9,77.7
N$309  (via drill 0.5)
  other vias: 79.7,77.7
N$310  (via drill 0.5)
  other vias: 78.5,77.7
N$311  (via drill 0.5)
  other vias: 77.3,77.7
N$312  (via drill 0.5)
  other vias: 76,77.7
N$313  (via drill 0.5)
  other vias: 74.8,77.7
N$314  (via drill 0.5)
  other vias: 73.6,77.7
N$315  (via drill 0.5)
  other vias: 71.2,77.7
N$316  (via drill 0.5)
  other vias: 69.9,77.7
N$317  (via drill 0.5)
  other vias: 67.9,90.2
N$318  (via drill 0.5)
  other vias: 69.2,90.2
N$319  (via drill 0.5)
  other vias: 70.5,90.2
N$320  (via drill 0.5)
  other vias: 71.8,90.2
N$321  (via drill 0.5)
  other vias: 73.1,90.2
N$322  (via drill 0.5)
  other vias: 74.4,90.2
N$323  (via drill 0.5)
  other vias: 74.4,88.9
N$324  (via drill 0.5)
  other vias: 73.1,88.9
N$325  (via drill 0.5)
  other vias: 71.7,88.9
N$326  (via drill 0.5)
  other vias: 70.4,88.9
N$327  (via drill 0.5)
  other vias: 69.1,88.9
N$328  (via drill 0.5)
  other vias: 67.9,89
N$329
  Bottom 1.27: 3.9,72.9 7.8,72.9
N$330
  Bottom 1.27: 18.1,68.8 16,68.8 16,87.3 | 16,87.3 16.7,87.3 | 16.7,87.3 17.8,87.3 17.8,69.5 17,69.5 17,69.7 16.8,69.7 16.8,87 16.7,87 16.7,87.3 | 16,87.3 10.3,87.3 10.3,91.7 10.2,91.7 10.2,94.6 9.8,94.6 9.8,92.2
N$331
  Top 1.27: 14.6,82.6 15.8,82.6 15.8,86.7 15.1,86.7 | 15,86.7 15.1,86.7 | 15.1,86.7 15.1,84.2 14.2,84.2 14.2,82.6
N$332  (3 unrouted)
  Top 1.27: U$3.3 30.4,79.9 30.4,80.2 30.3,80.2 30.2,84.8 30.2,86.3 | DPAK3.1 31.17,94 30.4,94 30.4,89.2 30.2,89.2 30.2,87 30.2,86.3 | PAD6.1 47,84.8 47,86.3 30.2,86.3
N$333  (4 unrouted)
  Top 0.406: 25.9,81.5 25.9,81.6 27.1,81.6 27.1,86.88 R42.1 24,86.88 24,94.8
  Top 1.27: U$3.2 25.1,81.6
N$334  (3 unrouted)
  Top 0.406: 79.5,96.56 79.5,97.39 | D6.C 44.6,81.7 57.1,81.7 57.1,99
  Top 1.27: DPAK3.4 40,91.9 40,99 57.1,99 65.4,99 65.4,99.1
  Top 3.81: 78.22,97.62 77.6,97 77.6,95.39 C18.+
N$335  (2 unrouted)
  Top 0.406: R35.1 44.3,77.34 44.3,77.5 | 45.35,77.45 46.7,76.1 46.7,74.5 50.1,71.1 69.7,71.1 74.3,74.6 77.1,74.6 80.05,72.55 80.05,70.35 80.4,70 88.8,70 | 45.35,77.45 45.3,77.5 | R34.1 92.38,71.08 91.4,70.1 88.9,70.1 | 45.35,77.45 44.51,77.45 R35.1 | U$3.5 25.6,76.5 25.6,71.9 42.9,71.9 42.9,76.9 44.2,76.9 | D6.A 44.51,79.7 R35.1
N$336  (via drill 0.5)  (12 unrouted)
  Top 0.406: 80,79.89 80,79.6 | Q3.E 22,68.34 22,68.5 | Q3.E 23.34,67.1 40,67.1 40.6,67.7 40.6,68.8 42.1,67.3 75.7,67.3 75.7,68.1 C19.2 | 14.2,83.3 14.4,83.3 14.4,82.9 | Q3.E 21.8,68 20.8,67.1 13.1,67.1 11.4,68.5 11.4,73.8 11.2,74 4.89,74 X5.2
  Top 1.27: 25.4,83.9 25.4,84.1 21.7,84.1 21.7,84 21.6,84 21.6,84.1 20.8,84.1 20.8,82.8 21.7,82.8 | R33.2 89.2,79.76 89.2,77.2 70.1,77.2 70.1,79.8 69.8,79.8 69.8,77.2 | 69.8,77.1 69.8,77.2 | 69.8,77.2 70.8,77.2 70.8,77.8 71.1,77.8 71.1,78.8 88.6,78.8 88.6,78.7 87.9,78.7 87.9,78 71.9,78 71.9,77.8 | D5.A 14.16,83.76 C20.2 14.4,86.42 14.4,83.3 | 14.4,82.9 15.2,82.9 v15.8,84.8 | C15.2 21.7,81.23 21.7,82.7 | 21.7,82.8 v21.7,83.3 v23,83.3 U$3.1 | 15.78,83.3 15.78,84.31 | 21.7,82.8 21.7,82.7 | 21.7,82.7 21.4,82.7 21.4,83.5
  Top 3.81: C18.- 68.9,89.97 68.9,91
  Bottom 1.27: 39.5,68.6 19.4,68.6 19.4,72 36.7,72 37.8,70.9 37.8,69.6 37.5,69.3 20.6,69.3 20.2,69.7 20.2,70.6 20.4,70.8 36.5,70.8 37.2,70.1 21.3,70.1 21.2,70 37.1,70 39,68.1 20.1,68.1 | 20.1,68.1 19.4,68.1 | 19.4,68.1 19.4,71.4 18.7,72.1 18.7,83.3 | 18.7,83.3 18.7,87.5 17.6,88.6 12.9,88.6 10.2,91.3 10.7,91.3 10.7,94.4 10.5,94.6 10.5,92.4 10.3,92.2 10.3,91.9 13,89.2 16.4,89.2 | 16.4,89.2 18.5,89.2 18.6,89.1 18.6,88.1 18.4,87.9 | 18.4,87.9 18.7,87.9 | 18.4,87.9 12.6,87.9 10.3,90.2 10.3,88.2 10.8,88.2 12,87 15,87 15.2,87.2 v15.8,84.8 | v15.8,84.8 15.2,68.1 15.3,68 20,68 20.1,68.1 | 19.4,68.1 18.8,68.1 18.5,68.4 18.5,71.3 18.6,71.4 | v15.8,84.8 15.7,86.7 15.7,84.7 | v21.7,83.3 v20.5,83.3 | v20.5,83.3 18.7,83.3 | C21.- 16.4,94.9 16.4,89.2 | v20.5,83.3 23.6,83.3 23.6,84.5 19.4,84.5
  Bottom 2.54: 85.2,77.3 86.9,77.3 86.9,76.5 89.6,76.5 89.6,90.7 68.3,90.7 68.3,91.3 68.5,91.3 68.5,88.6 69.6,88.6 69.6,86.9 69.5,86.9 69.5,80.6 42.6,80.6 42.6,80.9 | 42.4,80.9 42.4,77.8 87.9,77.8 87.9,89.3 71.39,89.3 | 69.3,89.3 71.39,89.3 | 71.39,89.3 R33.2 42.8,79.76 42.8,79.4 43.6,79.4 43.6,71.8 71.8,71.8 | 71.8,71.8 71.8,71.5 | 71.8,71.8 71.8,75.9 45.3,75.9 45.3,77.2 45.8,77.2 45.8,73.2 70.7,73.2 70.7,73.9 47,73.9 47,74.4 72.4,74.4 v72.4,77.7 72.4,88.5 85.6,88.5 85.6,87.3 86.5,87.3 86.5,80.3 74.4,80.3 | 74.4,80.3 74.4,79.49 | 74.4,80.3 74.4,87.3 84.9,87.3 84.9,85.7 85.4,85.7 85.4,81.3 75.6,81.3 75.6,81.1 76.1,81.1 76.1,85.2 83.3,85.2 83.3,84.8 83.5,84.8 83.5,83 77.9,83 77.9,82.8 83.4,82.8 83.4,71.1 80.4,71.1 | 80.4,71.1 80.4,70.9 | 80.4,71.1 80.4,75.9 81.9,75.9 | 82.5,75.9 81.9,75.9 | 81.9,75.9 81.9,71.5 | 84.7,69.2 85.6,69.2 85.6,68.1 78.3,68.1 78.3,68.6 78.4,68.6 78.4,69.7 82.5,69.7 82.5,69.2 78.1,69.2 78.1,70.3 39.5,70.3 39.5,68.6 73.2,68.6 73.2,69 73,69 73,69.2 | X5.2 4.46,74.5 7.9,74.5 8.7,75.3 8.7,98.6 7.2,98.6 7.7,98.1 7.7,67.8 8.7,67.8 8.8,67.9 8.8,74.7 8.01,75.49 C17.-
  Bottom 3.81: 84.7,69.2 84.7,69.4 85.2,69.4 85.2,77.3
N$337  (via drill 0.5)
  other vias: 20.5,84.5
N$338  (via drill 0.5)
  other vias: 21.7,84.5
N$339  (via drill 0.5)
  other vias: 23,84.5
N$340
  Top 1.27: 20.4,82.7 20.3,82.7 20.3,84.5 23.1,84.5 | 23.5,84.5 23.1,84.5 | 23.1,84.5 23.1,82.6 20.4,82.6
N$341  (via drill 0.5)
  Top 1.27: 18.6,78.8 18.7,78.8 18.7,99.1 2.2,99.1 2.2,99 0.7,99 0.7,98.8 0.6,98.8 v0.7,98 0.6,92.7 4.1,92.7 4.1,92.9 4.2,92.9 4.2,99.2 v3.1,99.2 v1.9,99.2 v0.7,99.2 0.6,99.2 0.6,99.1 1.8,99.1 v1.9,98 1.8,93.5
N$342  (via drill 0.5)
  Top 1.27: 4.7,98 v15.6,98 v16.8,98 17.9,98 17.9,97.9 17.6,97.9 17.6,96.8 v16.8,96.8 v15.6,96.8 4,96.8 4,97.1
  Bottom 1.27: 63.1,99 63.1,99.2 22.2,99.2 | 22.2,99 22.2,99.2 | 22.2,99.2 v18,99.2 v16.8,99.2 15.8,99.2 15.8,98.3 15.9,98.3 | 17.5,98.3 15.9,98.3 | 15.9,98.3 15.9,97.6 63.2,97.6 | 64.3,83.8 65.3,83.8 65.3,99.2 63.2,99.2 63.2,97.6 | 63.2,97.4 63.2,83.6 | 63.2,97.6 63.2,97.4 | 63.2,97.4 62.7,97.4 62.7,96.7 15.6,96.7 v15.6,96.8 v15.6,98 v15.6,99.2
N$343  (via drill 0.5)
  Top 1.27: 63.4,97.7 40.6,97.7 | 40.6,97.7 40.6,98.2 | 40.6,97.7 40.6,96.4 40.7,96.4 | 64.2,96.4 40.7,96.4 | 40.7,96.4 40.7,94.4 39.1,94.4 39.1,94.5 39.2,94.5 39.2,99 38.2,99 38.2,98.7 38.1,98.7 38.1,94.5 v35,94.6 33.8,94.5 33.8,99.2 73.7,99.2 73.7,99.1 35,99.1 35,95.4 37.1,95.4 37.1,97.9 36.1,97.9 | 36.1,97.9 36.1,98 | 36.1,97.9 36.1,96.2
N$344
  Top 1.27: 33.8,94.2 33.6,94.2 33.6,89.3 | 33.6,89.3 33.6,89.2 | 33.6,89.2 41.8,89.2 41.8,96.8 43,96.8 43,89 44.1,89 44.1,96.8 45.2,96.8 45.2,89 | 45.2,89 33.6,89 33.6,89.2 | 33.6,89.3 34.6,89.3 34.6,93.7 35.8,93.7 35.8,90.2 36.8,90.2 36.8,93.7 37,93.7 37,92.5 | 45.2,89 65.8,89 65.8,95.5 69.7,95.5 69.7,95.4 46.2,95.4 46.2,90 64.7,90 64.7,94.5 47.1,94.5 47.1,94.6 47.2,94.6 47.2,91.1 63.7,91.1 | 63.7,91.1 63.7,91 | 63.7,91.1 63.7,93.5 48.1,93.5 48.1,92.1 63,92.1 63,92.8 49,92.8 49,92.7
N$345
  Top 1.27: 45.5,97.1 62.8,97.1
N$346
  Top 1.27: 40.9,98.5 63.2,98.5 63.2,98.6
N$347
  Top 1.27: 31.6,93.9 31.7,93.9 31.7,90.3 31.4,90.3 31.4,85.5 32,85.5 32,94 30.9,94 30.9,91.2 29.4,91.2 29.4,94.3 29.3,94.3 29.3,85.2 29,85.2 29,94.4 32,94.4 32,94.3
N$348
  Top 1.27: 32.5,86.9 50.5,86.9 | 50.5,86.9 50.5,86.8 | 50.5,86.8 50.5,86.4 47.7,86.4 47.7,86.2 50.6,86.2 50.6,83.6 50.7,83.6 50.7,83.3 46.8,83.3 46.8,83.5 46.6,83.5 46.6,85.2 32.9,85.2 32.9,86.2 32.7,86.2 32.7,87.3 50.5,87.3 50.5,86.9 | 50.5,86.8 39.6,86.8 39.6,82.7 39.4,82.7 39.4,74.8 38.9,74.8 38.9,84.4 28.6,84.4 28.6,73.2 41.7,73.2 41.7,84.6 40.6,84.6 40.6,74 29.5,74 29.5,74.1
N$349
  Top 1.27: 19.3,78.8 23.1,78.8 23.1,77.5 18.2,77.5 18.2,77.6 17.7,77.6 17.7,77.8 17.6,77.8 17.6,81.8 17.5,81.8 17.5,96
N$350
  Top 1.27: 16.6,96.4 16.6,88.7 16.9,88.7 16.9,88.8
N$351
  Top 1.27: 18.6,99 18.8,99 18.8,99.1
N$352  (via drill 0.5)
  Top 1.27: 32,94.5 32,99.2 25.7,99.2 25.7,94.1 25.8,94.1 25.8,88.3 v27.1,88.3 28.4,88.3 28.4,88.2 26.7,88.2 26.7,98.2 31.1,98.2 31.1,95.5 27.8,95.5 27.8,89.2 28.4,89.2 v28.4,89.6 v28.4,90.9 v28.4,92.2 v28.4,93.5 v28.4,94.8 28.4,97.3 27.6,97.3 27.6,96.2 30.2,96.2 30.2,96.3 29.2,96.3 29.2,97.3 30.3,97.3 30.3,97.1
N$353  (via drill 0.5)
  other vias: 3.2,98
N$354  (via drill 0.5)
  other vias: 0.7,96.8
N$355  (via drill 0.5)
  other vias: 1.9,96.8
N$356  (via drill 0.5)
  other vias: 3.2,96.8
N$357  (via drill 0.5)
  other vias: 18,98
N$358  (via drill 0.5)
  other vias: 18.1,96.8
N$359  (via drill 0.5)
  other vias: 28.7,73.7
N$360  (via drill 0.5)
  other vias: 29.9,73.7
N$361  (via drill 0.5)
  other vias: 31.1,73.7
N$362  (via drill 0.5)
  other vias: 32.3,73.7
N$363  (via drill 0.5)
  other vias: 33.5,73.7
N$364  (via drill 0.5)
  other vias: 34.7,73.7
N$365  (via drill 0.5)
  other vias: 35.9,73.7
N$366  (via drill 0.5)
  other vias: 37.1,73.7
N$367  (via drill 0.5)
  other vias: 38.3,73.7
N$368  (via drill 0.5)
  other vias: 39.5,73.7
N$369  (via drill 0.5)
  other vias: 40.7,73.7
N$370  (via drill 0.5)
  other vias: 39.9,75
N$371  (via drill 0.5)
  other vias: 41.2,75
N$372  (via drill 0.5)
  other vias: 40.2,77.6
N$373  (via drill 0.5)
  other vias: 40.2,78.8
N$374  (via drill 0.5)
  other vias: 40.2,80.1
N$375  (via drill 0.5)
  other vias: 40.2,81.4
N$376  (via drill 0.5)
  other vias: 40.2,82.7
N$377  (via drill 0.5)
  other vias: 40.2,84
N$378  (via drill 0.5)
  other vias: 29.2,85.9
N$379  (via drill 0.5)
  other vias: 30.4,85.9
N$380  (via drill 0.5)
  other vias: 31.6,85.9
N$381  (via drill 0.5)
  other vias: 32.8,85.9
N$382  (via drill 0.5)
  other vias: 34,85.9
N$383  (via drill 0.5)
  other vias: 35.2,85.9
N$384  (via drill 0.5)
  other vias: 36.4,85.9
N$385  (via drill 0.5)
  other vias: 37.6,85.9
N$386  (via drill 0.5)
  other vias: 38.8,85.9
N$387  (via drill 0.5)
  other vias: 40,85.9
N$388  (via drill 0.5)
  other vias: 29.2,87.1
N$389  (via drill 0.5)
  other vias: 30.4,87.1
N$390  (via drill 0.5)
  other vias: 31.6,87.1
N$391  (via drill 0.5)
  other vias: 32.8,87.1
N$392  (via drill 0.5)
  other vias: 34,87.1
N$393  (via drill 0.5)
  other vias: 35.2,87.1
N$394  (via drill 0.5)
  other vias: 36.4,87.1
N$395  (via drill 0.5)
  other vias: 37.6,87.1
N$396  (via drill 0.5)
  other vias: 38.8,87.1
N$397  (via drill 0.5)
  other vias: 40,87.2
N$398  (via drill 0.5)
  other vias: 41.2,87.1
N$399  (via drill 0.5)
  other vias: 41.2,85.9
N$400  (via drill 0.5)
  other vias: 41.4,84.4
N$401  (via drill 0.5)
  other vias: 41.5,83.1
N$402  (via drill 0.5)
  other vias: 28.4,88.4
N$403  (via drill 0.5)
  other vias: 27.1,94.8
N$404  (via drill 0.5)
  other vias: 27.1,93.6
N$405  (via drill 0.5)
  other vias: 27.1,92.2
N$406  (via drill 0.5)
  other vias: 27.1,90.9
N$407  (via drill 0.5)
  other vias: 27.1,89.5
N$408  (via drill 0.5)
  other vias: 42.5,89.3
N$409  (via drill 0.5)
  other vias: 42.5,90.6
N$410  (via drill 0.5)
  other vias: 42.5,91.9
N$411  (via drill 0.5)
  other vias: 42.5,93.2
N$412  (via drill 0.5)
  other vias: 42.5,94.5
N$413  (via drill 0.5)
  other vias: 43.8,94.5
N$414  (via drill 0.5)
  other vias: 43.8,93.2
N$415  (via drill 0.5)
  other vias: 43.7,91.9
N$416  (via drill 0.5)
  other vias: 43.7,90.6
N$417  (via drill 0.5)
  other vias: 43.7,89.3
N$418  (via drill 0.5)
  Bottom 1.27: 34,95 v37.5,95 v38.7,95 v40.1,95 v41.3,95 61.4,95 61.4,89 33.9,89 33.9,95 34.7,95 34.7,89.6
N$419
  Bottom 1.27: 35.3,89.8 60.6,89.8 60.6,94 35.6,94 35.6,90.9 59.7,90.9 59.7,93.1 36.6,93.1 36.6,91.9
N$420
  Bottom 1.27: 37.3,91.8 59.2,91.8 59.2,92.1 37.6,92.1 37.6,92.8
N$421  (via drill 0.5)
  Bottom 1.27: 25.8,94.8 25.7,94.8 | 25.7,94.8 25.7,94.9 | 25.7,94.9 25.7,95.1 32,95.1 32,86.8 32.8,86.8 32.8,87.3 50.5,87.3 50.5,87 50.6,87 50.6,83.3 41.7,83.3 41.7,84.1 41.4,84.1 41.4,86.5 49.7,86.5 49.7,86 42.7,86 42.7,84.1 49.6,84.1 49.6,85.2 43.7,85.2 43.7,85.1 40.5,85.1 40.5,82.4 40.3,82.4 40.3,81.7 40.1,81.7 v40.1,76.3 40.1,75.5 41.3,75.5 41.3,73.7 25.7,73.7 25.7,94.8 | 25.7,94.9 31,94.9 31,86.7 26.3,86.7 26.3,87.4 26.5,87.4 26.5,94.3 30.1,94.3 30.1,87.7 27.4,87.7 27.4,93.8 29,93.8 29,88.2 28.1,88.2 28.1,93.1
N$422
  Bottom 1.27: 26.4,85.7 40.8,85.7 40.8,86.5 34,86.5 34,86.4 39.3,86.4 39.3,73.9 40.3,73.9 40.3,74.5 26.8,74.5 26.8,84.8 39,84.8 39,75 27.5,75 27.5,83.9 37.9,83.9 37.9,75.7 28.5,75.7 28.5,82.9 36.8,82.9 36.8,76.6 29.4,76.6 29.4,82 35.6,82 35.6,77.4 30.3,77.4 30.3,81.3 34.5,81.3 34.5,78.4 31.3,78.4 31.3,80.3 33.5,80.3 33.5,79.2 32.2,79.2 32.2,79.4
N$423
  Bottom 1.27: 37.5,71.6 43,71.6 43,71.7 42.5,71.7 | 42.5,71.7 37,71.7 | 37,71.7 37,71.9 42.5,71.9 42.5,71.7 | 37,71.7 19.3,71.7 19.3,89.6 12.1,89.6 12.1,89.5
N$424
  Top 0.406: 23.6,94.9 23.7,94.9 23.7,87.2 22.8,87.2
N$425
  Bottom 0.406: 25.6,73.3 20.5,73.3 20.5,81.9 25.1,81.9 25.1,73.6 20.8,73.6 20.8,81.7 24.8,81.7 24.8,81.4 24.7,81.4 24.7,73.9 21.2,73.9 21.2,74 21,74 21,81.5 24.4,81.5 24.4,74.3 21.3,74.3 21.3,81.3 24,81.3 24,74.6 21.6,74.6 21.6,81.1 23.7,81.1 23.7,74.9 21.9,74.9 21.9,80.9 23.4,80.9 23.4,75 22.3,75 22.3,80.6 23.1,80.6 23.1,75.3 22.7,75.3 22.7,80.4 22.4,80.4 22.4,79.7
N$426
  Bottom 0.406: 25.3,85.9 25,85.9 25,82.2 24.9,82.2 24.9,85.8 20.6,85.8 20.6,86.6 20.7,86.6 20.7,93.2 25.1,93.2 25.1,92.7 24.9,92.7 24.9,93 25,93 25,86.1 20.9,86.1 20.9,86.4 21,86.4 21,92.8 24.7,92.8 24.7,86.4 21.3,86.4 21.3,92.4 24.4,92.4 24.4,86.7 21.7,86.7 21.7,92.1 24,92.1 24,86.9 22.1,86.9 22.1,91.8 23.7,91.8 23.7,87.2 22.5,87.2 22.5,91.5 23.4,91.5 23.4,87.4 22.9,87.4 22.9,91.2
N$427  (via drill 0.5)
  other vias: 36.2,89.5
N$428  (via drill 0.5)
  other vias: 36.2,90.8
N$429  (via drill 0.5)
  other vias: 36.2,92.1
N$430  (via drill 0.5)
  other vias: 36.3,93.3
N$431  (via drill 0.5)
  other vias: 36.3,94.6
N$432  (via drill 0.5)
  other vias: 34.8,89.5
N$433  (via drill 0.5)
  other vias: 34.8,90.8
N$434  (via drill 0.5)
  other vias: 34.9,92.1
N$435  (via drill 0.5)
  other vias: 35,93.3
S$1
  Bottom 0.406: 0.3,68.9 0.2,68.9 0.2,65.6 4.5,65.6 4.5,66.6 0.5,66.6 0.5,68.5 1.1,68.5 1.1,67 0.8,67 0.8,68.1
S$2
  Bottom 0.406: 6.7,67.5 6.6,67.5 6.6,66.4 6.8,66.4 6.8,66.7 7.3,66.7 7.3,66.6 9.9,66.6 | 9.9,66.6 9.9,67.8 | 9.9,66.6 9.9,62 9.6,62 9.6,67
S$3
  Bottom 0.406: 0.2,35.8 0.2,32.5 0.6,32.5 0.6,35.1 0.9,35.1 0.9,33.3 1.3,33.3 1.3,34.8 2,34.8 2,33.3 4.6,33.3 | 4.7,33.3 4.6,33.3 | 4.6,33.3 4.6,32.5 4.4,32.5 4.4,33
S$4
  Bottom 0.406: 6.7,34.5 6.7,33.1 7,33.1 7,33.5 7.2,33.5 7.2,33.3 9.7,33.3 9.7,32.5 9.9,32.5 | 9.9,32.5 9.9,34.6 | 9.9,32.5 9.9,28.3 9.6,28.3 9.6,33.7
S$5
  Bottom 0.406: 1.3,0.3 0.2,0.3 0.2,2.6 0.5,2.6 0.5,0.6 1.1,0.6 1.1,1.5 0.8,1.5 0.8,0.8
S$6
  Bottom 1.27: 7.5,42.8 3.9,42.8
S$7
  Bottom 1.016: 2.5,49.3 2.4,49.3
S$8
  Bottom 2.54: 4.46,41.2 7.9,41.2 8.7,42 8.7,65.3 7.2,65.3 7.7,64.8 7.7,34.5 8.7,34.5 8.8,34.6 8.8,41.4 8.01,42.19 C10.-
S$9
  Bottom 0.406: 3.4,43.2 3.4,39.2 3.6,39.2 3.6,43.2
S$10
  Bottom 0.406: 2.7,48.8 4.6,48.8 4.6,49.7 4.3,49.7 4.3,49.1 2.5,49.1 2.5,37.8
S$11
  Bottom 1.27: 7.5,9.5 3.9,9.5
S$12
  Bottom 1.016: 2.5,16 2.4,16
S$13
  Bottom 0.406: 3.5,9.9 3.5,5.9 3.8,5.9 3.8,6.1
S$14
  Bottom 0.406: 2.6,4.6 2.5,4.6 2.5,15.5 4.6,15.5 4.6,16.8 4.2,16.8 4.2,15.6
S$15
  Bottom 1.27: 7.5,76.1 3.9,76.1
S$16
  Bottom 1.016: 2.5,82.6 2.4,82.6
S$17
  Bottom 0.406: 3.7,76.2 3.5,76.2 3.5,76.5 3.4,76.5 3.4,72.5 3.7,72.5 | 3.8,72.5 3.7,72.5 | 3.7,72.5 3.7,75.6
S$18
  Bottom 0.406: 2.6,71.1 2.5,71.1 2.5,82.1 4.6,82.1 4.6,83.3 4.3,83.3 4.3,82.2

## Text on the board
tNames: A + | K - | Dim | - | + | A + | K - | Dim | - | + | A + | K - | Dim | - | +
